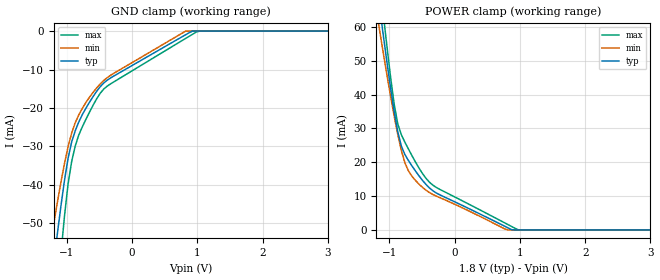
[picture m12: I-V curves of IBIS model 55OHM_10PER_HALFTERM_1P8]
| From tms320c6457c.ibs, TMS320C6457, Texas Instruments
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|   Model Cell 55OHM_10PER_HALFTERM_1P8
|55OHM_10PER_HALFTERM_1P8
[Model]   55OHM_10PER_HALFTERM_1P8
Model_type   Input
Polarity   Non-Inverting
Vinl =  0.8
Vinh =  1
C_comp   1.89p   1.72p   2.18p
[Model Spec]
Vinl   0.8   0.71   0.89
Vinh   1   0.91   1.09
D_overshoot_high 2.34 NA NA
D_overshoot_low -0.54 NA NA
D_overshoot_time 0.56n NA NA
S_overshoot_high 2.2 NA NA
S_overshoot_low -0.4 NA NA
[Receiver Thresholds]
Vth = 0.9V
Vth_min = 0.855V
Vth_max = 0.945V
Vinl_dc = -125mV
Vinh_dc = +125mV
Vinl_ac = -250mV
Vinh_ac = +250mV
Tslew_ac = 5.000ns
Threshold_sensitivity = 0.50
Reference_supply Pullup_ref
[Temperature Range]   25   125   -40
[Voltage Range]   1.8   1.62   1.98
[Pullup reference]   1.8   1.62   1.98
[POWER_clamp]
|   voltage   I(typ)   I(min)   I(max)
-1.8V     165.8mA    141.3mA    194.3mA
-1.145V   65.14mA    58.47mA    73.04mA
-1.091V   57.19mA    52.01mA    63.42mA
-1.036V   49.44mA    45.69mA    54.07mA
-927.3mV  35.09mA    33.73mA    37.29mA
-872.7mV  29.14mA    28.32mA    31.45mA
-818.2mV  24.87mA    23.61mA    28.2mA
-654.5mV  18.95mA    15.87mA    21.97mA
-381.8mV  12.34mA    10.99mA    14.04mA
763.6mV   1.139mA    347.9uA    2.133mA
981.8mV   0A         0A         0A
3.6V      0A         0A         0A
[GND_clamp]
|   voltage   I(typ)   I(min)   I(max)
-1.8V     -153mA     -119.3mA   -208.2mA
-1.255V   -67.89mA   -55.76mA   -90.57mA
-1.2V     -60.17mA   -50.02mA   -79.42mA
-1.145V   -52.68mA   -44.53mA   -68.5mA
-1.091V   -45.49mA   -39.31mA   -57.93mA
-1.036V   -38.82mA   -34.45mA   -48.09mA
-981.8mV  -33.11mA   -30.12mA   -39.81mA
-872.7mV  -25.97mA   -23.89mA   -29.95mA
-490.9mV  -14.51mA   -13.8mA    -16.23mA
818.2mV   -967.9uA   -29.76uA   -1.925mA
1.036V    0A         0A         0A
3.6V      0A         0A         0A
